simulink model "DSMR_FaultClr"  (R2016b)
settings: Solver=FixedStepDiscrete  StartTime=0.0  StopTime=10.0  FixedStep=0.01  RelTol=1e-3  EnableMultiTasking=on
undefined symbols (not defined in the file): bin2dec, DSMAUX_xClearTrg_C
libraries: simulink x156

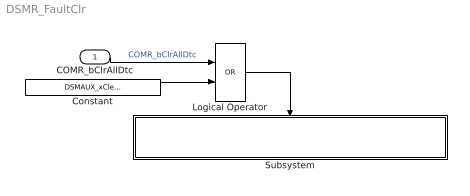
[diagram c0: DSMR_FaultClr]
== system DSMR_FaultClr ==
  COMR_bClrAllDtc : Inport
  Constant : Constant  Value=DSMAUX_xClearTrg_C
  Logical Operator : Logic  Operator=OR  AllPortsSameDT=off  OutDataTypeStr=boolean
  Subsystem : Subsystem
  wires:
  Constant/1 -> Logical Operator/2
  COMR_bClrAllDtc/1 -> Logical Operator/1  "COMR_bClrAllDtc"
  Logical Operator/1 -> Subsystem/Trigger

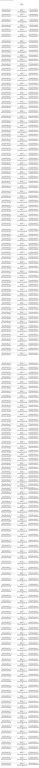
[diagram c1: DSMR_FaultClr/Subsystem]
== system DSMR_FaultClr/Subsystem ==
  Trigger : TriggerPort  VariantControl=Variant  PortDimensions=1
  Bitwise Operator{1..156} (156 alike) : simulink/Logic and Bit Operations/Bitwise Operator  logicop=AND  UseBitMask=on  BitMask=bin2dec('00000000')  BitMaskRealWorld=Stored Integer
  Data Store Read : DataStoreRead  DataStoreName=DFC_CurrRngErr
  Data Store Read1 : DataStoreRead  DataStoreName=DFC_BattVoltRngErr
  Data Store Read10 : DataStoreRead  DataStoreName=DFC_RcMsg2A3Mis
  Data Store Read100 : DataStoreRead  DataStoreName=DFC_CC2Chk
  Data Store Read101 : DataStoreRead  DataStoreName=DFC_APlusChk
  Data Store Read102 : DataStoreRead  DataStoreName=DFC_DChrgMsgTmt
  Data Store Read103 : DataStoreRead  DataStoreName=DFC_DChrgTNegElecMax
  Data Store Read104 : DataStoreRead  DataStoreName=DFC_DChrgTNegElecMin
  Data Store Read105 : DataStoreRead  DataStoreName=DFC_DChrgTNegElecSig
  Data Store Read106 : DataStoreRead  DataStoreName=DFC_DChrgTPosElecMax
  Data Store Read107 : DataStoreRead  DataStoreName=DFC_DChrgTPosElecMin
  Data Store Read108 : DataStoreRead  DataStoreName=DFC_DChrgTPosElecSig
  Data Store Read109 : DataStoreRead  DataStoreName=DFC_CcuSelfChkErr
  Data Store Read11 : DataStoreRead  DataStoreName=DFC_ChkSumMsg2A3Err
  Data Store Read110 : DataStoreRead  DataStoreName=DFC_ChrgOCMin
  Data Store Read111 : DataStoreRead  DataStoreName=DFC_ChrgOCMax
  Data Store Read112 : DataStoreRead  DataStoreName=DFC_DisChOCMax
  Data Store Read113 : DataStoreRead  DataStoreName=DFC_SocRngLoMax
  Data Store Read114 : DataStoreRead  DataStoreName=DFC_SocRngLoMin
  Data Store Read115 : DataStoreRead  DataStoreName=DFC_SocRngHiMax
  Data Store Read116 : DataStoreRead  DataStoreName=DFC_SocRngHiMin
  Data Store Read117 : DataStoreRead  DataStoreName=DFC_InClntOverTmp
  Data Store Read118 : DataStoreRead  DataStoreName=DFC_OutClntOverTmp
  Data Store Read119 : DataStoreRead  DataStoreName=DFC_ClntDsTElecMax
  Data Store Read12 : DataStoreRead  DataStoreName=DFC_RcMsg2A5Mis
  Data Store Read120 : DataStoreRead  DataStoreName=DFC_ClntDsTElecMin
  Data Store Read121 : DataStoreRead  DataStoreName=DFC_ClntDsTElecSig
  Data Store Read122 : DataStoreRead  DataStoreName=DFC_ClntUsTElecMax
  Data Store Read123 : DataStoreRead  DataStoreName=DFC_ClntUsTElecMin
  Data Store Read124 : DataStoreRead  DataStoreName=DFC_ClntUsTElecSig
  Data Store Read125 : DataStoreRead  DataStoreName=DFC_CoolPerfPlaus
  Data Store Read126 : DataStoreRead  DataStoreName=DFC_HtgPerfPlaus
  Data Store Read127 : DataStoreRead  DataStoreName=DFC_DChrgFobd
  Data Store Read128 : DataStoreRead  DataStoreName=DFC_DChrgHvOnFail
  Data Store Read129 : DataStoreRead  DataStoreName=DFC_AChgHVOnTmt
  Data Store Read13 : DataStoreRead  DataStoreName=DFC_RcMsg2A7Mis
  Data Store Read130 : DataStoreRead  DataStoreName=DFC_AChgHVOffTmt
  Data Store Read131 : DataStoreRead  DataStoreName=DFC_AChgS2ClsdTmt
  Data Store Read132 : DataStoreRead  DataStoreName=DFC_DChrgStakeErr
  Data Store Read133 : DataStoreRead  DataStoreName=DFC_DChrgStkVoltErr
  Data Store Read134 : DataStoreRead  DataStoreName=DFC_DChrgStkCurrErr
  Data Store Read135 : DataStoreRead  DataStoreName=DFC_AChgPileRdyTmt
  Data Store Read136 : DataStoreRead  DataStoreName=DFC_DChrgCHMTmt
  Data Store Read137 : DataStoreRead  DataStoreName=DFC_DChrgCRMTmt
  Data Store Read138 : DataStoreRead  DataStoreName=DFC_DChrgCMLTmt
  Data Store Read139 : DataStoreRead  DataStoreName=DFC_DChrgCROTmt
  Data Store Read14 : DataStoreRead  DataStoreName=DFC_MPosStuckMin
  Data Store Read140 : DataStoreRead  DataStoreName=DFC_DChrgCCSTmt
  Data Store Read141 : DataStoreRead  DataStoreName=DFC_DChrgCSTTmt
  Data Store Read142 : DataStoreRead  DataStoreName=DFC_DChrgCSDTmt
  Data Store Read143 : DataStoreRead  DataStoreName=DFC_DChrgParaChk
  Data Store Read144 : DataStoreRead  DataStoreName=DFC_DChrgCableChk
  Data Store Read145 : DataStoreRead  DataStoreName=DFC_DChrgSLACTOut
  Data Store Read146 : DataStoreRead  DataStoreName=DFC_DChrgCnntErr
  Data Store Read147 : DataStoreRead  DataStoreName=DFC_DChrgLckErr
  Data Store Read148 : DataStoreRead  DataStoreName=DFC_AChrgCnntErr
  Data Store Read149 : DataStoreRead  DataStoreName=DFC_AChgLckTmt
  Data Store Read15 : DataStoreRead  DataStoreName=DFC_MNegStuckMax
  Data Store Read150 : DataStoreRead  DataStoreName=DFC_AChgRdyPndiTmt
  Data Store Read151 : DataStoreRead  DataStoreName=DFC_AChgRdyTmt
  Data Store Read152 : DataStoreRead  DataStoreName=DFC_AChgingErr
  Data Store Read153 : DataStoreRead  DataStoreName=DFC_AChgUnlckTmt
  Data Store Read154 : DataStoreRead  DataStoreName=DFC_AChgFobd
  Data Store Read155 : DataStoreRead  DataStoreName=DFC_SocValJmp
  Data Store Read16 : DataStoreRead  DataStoreName=DFC_MNegStuckMin
  Data Store Read17 : DataStoreRead  DataStoreName=DFC_PrStuckMin
  Data Store Read18 : DataStoreRead  DataStoreName=DFC_CrashNpl
  Data Store Read19 : DataStoreRead  DataStoreName=DFC_FuseNpl
  Data Store Read2 : DataStoreRead  DataStoreName=DFC_BattHVMsgTmt
  Data Store Read20 : DataStoreRead  DataStoreName=DFC_Kl30cVoltLoErr
  Data Store Read21 : DataStoreRead  DataStoreName=DFC_PosStuckMax
  Data Store Read22 : DataStoreRead  DataStoreName=DFC_HvPwrUpFail
  Data Store Read23 : DataStoreRead  DataStoreName=DFC_DChrgPwrUpFail
  Data Store Read24 : DataStoreRead  DataStoreName=DFC_BattTAlrmMax
  Data Store Read25 : DataStoreRead  DataStoreName=DFC_BattTFaultMax
  Data Store Read26 : DataStoreRead  DataStoreName=DFC_DChrgPosStuckMax
  Data Store Read27 : DataStoreRead  DataStoreName=DFC_DChrgPosStuckMin
  Data Store Read28 : DataStoreRead  DataStoreName=DFC_DChrgNegStuckMax
  Data Store Read29 : DataStoreRead  DataStoreName=DFC_DChrgNegStuckMin
  Data Store Read3 : DataStoreRead  DataStoreName=DFC_BusHVMsgTmt
  Data Store Read30 : DataStoreRead  DataStoreName=DFC_BattTGradtMax
  Data Store Read31 : DataStoreRead  DataStoreName=DFC_CellVoltAlrmMax
  Data Store Read32 : DataStoreRead  DataStoreName=DFC_CellVoltFaultMax
  Data Store Read33 : DataStoreRead  DataStoreName=DFC_CellVoltFusfMax
  Data Store Read34 : DataStoreRead  DataStoreName=DFC_BattTAlrmMin
  Data Store Read35 : DataStoreRead  DataStoreName=DFC_BattTFaultMin
  Data Store Read36 : DataStoreRead  DataStoreName=DFC_BattTempVldMin
  Data Store Read37 : DataStoreRead  DataStoreName=DFC_BattTCnstMax
  Data Store Read38 : DataStoreRead  DataStoreName=DFC_CellVoltNpl
  Data Store Read39 : DataStoreRead  DataStoreName=DFC_Msg2E6Tmt
  Data Store Read4 : DataStoreRead  DataStoreName=DFC_638LinCommErr
  Data Store Read40 : DataStoreRead  DataStoreName=DFC_RcMsg2E0Mis
  Data Store Read41 : DataStoreRead  DataStoreName=DFC_ChkSumMsg2E0Err
  Data Store Read42 : DataStoreRead  DataStoreName=DFC_CellVoltAlrmMin
  Data Store Read43 : DataStoreRead  DataStoreName=DFC_CellVoltFusfMin
  Data Store Read44 : DataStoreRead  DataStoreName=DFC_CellVoltFaultMin
  Data Store Read45 : DataStoreRead  DataStoreName=DFC_CellVoltVldMin
  Data Store Read46 : DataStoreRead  DataStoreName=DFC_ChrgOCNpl
  Data Store Read47 : DataStoreRead  DataStoreName=DFC_DisChOCNpl
  Data Store Read48 : DataStoreRead  DataStoreName=DFC_BattVoltHiMax
  Data Store Read49 : DataStoreRead  DataStoreName=DFC_BattVoltLoMin
  Data Store Read5 : DataStoreRead  DataStoreName=DFC_CellTempTmt
  Data Store Read50 : DataStoreRead  DataStoreName=DFC_RcMsg2E1Mis
  Data Store Read51 : DataStoreRead  DataStoreName=DFC_ChkSumMsg2E1Err
  Data Store Read52 : DataStoreRead  DataStoreName=DFC_DcCanBusOff
  Data Store Read53 : DataStoreRead  DataStoreName=DFC_DChrgTCnntMax
  Data Store Read54 : DataStoreRead  DataStoreName=DFC_CurrChrgPlaus
  Data Store Read55 : DataStoreRead  DataStoreName=DFC_BattUNpl
  Data Store Read56 : DataStoreRead  DataStoreName=DFC_BattVoltVld
  Data Store Read57 : DataStoreRead  DataStoreName=DFC_PackUNpl
  Data Store Read58 : DataStoreRead  DataStoreName=DFC_ThmRnwy
  Data Store Read59 : DataStoreRead  DataStoreName=DFC_AChrgPortOvrTemp
  Data Store Read6 : DataStoreRead  DataStoreName=DFC_CellVoltTmt
  Data Store Read60 : DataStoreRead  DataStoreName=DFC_CurrOffsPlaus
  Data Store Read61 : DataStoreRead  DataStoreName=DFC_CurrStukPlaus
  Data Store Read62 : DataStoreRead  DataStoreName=DFC_EepReadErr
  Data Store Read63 : DataStoreRead  DataStoreName=DFC_BalStuckMax
  Data Store Read64 : DataStoreRead  DataStoreName=DFC_DChrgVoltVld
  Data Store Read65 : DataStoreRead  DataStoreName=DFC_BoardTempTmt
  Data Store Read66 : DataStoreRead  DataStoreName=DFC_PackVoltVld
  Data Store Read67 : DataStoreRead  DataStoreName=DFC_BalStuckMin
  Data Store Read68 : DataStoreRead  DataStoreName=DFC_CSCPwrSpyHiErr
  Data Store Read69 : DataStoreRead  DataStoreName=DFC_DChrgUNpl
  Data Store Read7 : DataStoreRead  DataStoreName=DFC_InCanBusOff
  Data Store Read70 : DataStoreRead  DataStoreName=DFC_HvilMax
  Data Store Read71 : DataStoreRead  DataStoreName=DFC_HvilMin
  Data Store Read72 : DataStoreRead  DataStoreName=DFC_HvilSig
  Data Store Read73 : DataStoreRead  DataStoreName=DFC_ChkSumMsg050Err
  Data Store Read74 : DataStoreRead  DataStoreName=DFC_RcMsg050Mis
  Data Store Read75 : DataStoreRead  DataStoreName=DFC_CrashHwNpl
  Data Store Read76 : DataStoreRead  DataStoreName=DFC_IsoChkLv1
  Data Store Read77 : DataStoreRead  DataStoreName=DFC_IsoChkLv2
  Data Store Read78 : DataStoreRead  DataStoreName=DFC_DisChOCMin
  Data Store Read79 : DataStoreRead  DataStoreName=DFC_InsResValdFault
  Data Store Read8 : DataStoreRead  DataStoreName=DFC_VeCanBusOff
  Data Store Read80 : DataStoreRead  DataStoreName=DFC_Kl30OutRngErr
  Data Store Read81 : DataStoreRead  DataStoreName=DFC_Kl30VoltLoErr
  Data Store Read82 : DataStoreRead  DataStoreName=DFC_Kl30VoltHiErr
  Data Store Read83 : DataStoreRead  DataStoreName=DFC_CSCPwrSpyLoErr
  Data Store Read84 : DataStoreRead  DataStoreName=DFC_CmcBordOTMax
  Data Store Read85 : DataStoreRead  DataStoreName=DFC_BattTWarnMax
  Data Store Read86 : DataStoreRead  DataStoreName=DFC_BattTWarnMin
  Data Store Read87 : DataStoreRead  DataStoreName=DFC_BattTempVldMax
  Data Store Read88 : DataStoreRead  DataStoreName=DFC_BattTHopMax
  Data Store Read89 : DataStoreRead  DataStoreName=DFC_CellVoltRngHiErr
  Data Store Read9 : DataStoreRead  DataStoreName=DFC_Msg2A3Tmt
  Data Store Read90 : DataStoreRead  DataStoreName=DFC_CellVoltRngLoErr
  Data Store Read91 : DataStoreRead  DataStoreName=DFC_CellVoltWarnMax
  Data Store Read92 : DataStoreRead  DataStoreName=DFC_CellVoltWarnMin
  Data Store Read93 : DataStoreRead  DataStoreName=DFC_CellVoltVldMax
  Data Store Read94 : DataStoreRead  DataStoreName=DFC_AChrgCurrMish
  Data Store Read95 : DataStoreRead  DataStoreName=DFC_DChrgCurrMish
  Data Store Read96 : DataStoreRead  DataStoreName=DFC_DChrgLowTempCurrMish
  Data Store Read97 : DataStoreRead  DataStoreName=DFC_AChrgVoltMish
  Data Store Read98 : DataStoreRead  DataStoreName=DFC_DChrgVoltMish
  Data Store Read99 : DataStoreRead  DataStoreName=DFC_DChrgBattTMin
  Data Store Write : DataStoreWrite  DataStoreName=DFC_CurrRngErr
  Data Store Write1 : DataStoreWrite  DataStoreName=DFC_BattVoltRngErr
  Data Store Write10 : DataStoreWrite  DataStoreName=DFC_RcMsg2A3Mis
  Data Store Write100 : DataStoreWrite  DataStoreName=DFC_CC2Chk
  Data Store Write101 : DataStoreWrite  DataStoreName=DFC_APlusChk
  Data Store Write102 : DataStoreWrite  DataStoreName=DFC_DChrgMsgTmt
  Data Store Write103 : DataStoreWrite  DataStoreName=DFC_DChrgTNegElecMax
  Data Store Write104 : DataStoreWrite  DataStoreName=DFC_DChrgTNegElecMin
  Data Store Write105 : DataStoreWrite  DataStoreName=DFC_DChrgTNegElecSig
  Data Store Write106 : DataStoreWrite  DataStoreName=DFC_DChrgTPosElecMax
  Data Store Write107 : DataStoreWrite  DataStoreName=DFC_DChrgTPosElecMin
  Data Store Write108 : DataStoreWrite  DataStoreName=DFC_DChrgTPosElecSig
  Data Store Write109 : DataStoreWrite  DataStoreName=DFC_CcuSelfChkErr
  Data Store Write11 : DataStoreWrite  DataStoreName=DFC_ChkSumMsg2A3Err
  Data Store Write110 : DataStoreWrite  DataStoreName=DFC_ChrgOCMin
  Data Store Write111 : DataStoreWrite  DataStoreName=DFC_ChrgOCMax
  Data Store Write112 : DataStoreWrite  DataStoreName=DFC_DisChOCMax
  Data Store Write113 : DataStoreWrite  DataStoreName=DFC_SocRngLoMax
  Data Store Write114 : DataStoreWrite  DataStoreName=DFC_SocRngLoMin
  Data Store Write115 : DataStoreWrite  DataStoreName=DFC_SocRngHiMax
  Data Store Write116 : DataStoreWrite  DataStoreName=DFC_SocRngHiMin
  Data Store Write117 : DataStoreWrite  DataStoreName=DFC_InClntOverTmp
  Data Store Write118 : DataStoreWrite  DataStoreName=DFC_OutClntOverTmp
  Data Store Write119 : DataStoreWrite  DataStoreName=DFC_ClntDsTElecMax
  Data Store Write12 : DataStoreWrite  DataStoreName=DFC_RcMsg2A5Mis
  Data Store Write120 : DataStoreWrite  DataStoreName=DFC_ClntDsTElecMin
  Data Store Write121 : DataStoreWrite  DataStoreName=DFC_ClntDsTElecSig
  Data Store Write122 : DataStoreWrite  DataStoreName=DFC_ClntUsTElecMax
  Data Store Write123 : DataStoreWrite  DataStoreName=DFC_ClntUsTElecMin
  Data Store Write124 : DataStoreWrite  DataStoreName=DFC_ClntUsTElecSig
  Data Store Write125 : DataStoreWrite  DataStoreName=DFC_CoolPerfPlaus
  Data Store Write126 : DataStoreWrite  DataStoreName=DFC_HtgPerfPlaus
  Data Store Write127 : DataStoreWrite  DataStoreName=DFC_DChrgFobd
  Data Store Write128 : DataStoreWrite  DataStoreName=DFC_DChrgHvOnFail
  Data Store Write129 : DataStoreWrite  DataStoreName=DFC_AChgHVOnTmt
  Data Store Write13 : DataStoreWrite  DataStoreName=DFC_RcMsg2A7Mis
  Data Store Write130 : DataStoreWrite  DataStoreName=DFC_AChgHVOffTmt
  Data Store Write131 : DataStoreWrite  DataStoreName=DFC_AChgS2ClsdTmt
  Data Store Write132 : DataStoreWrite  DataStoreName=DFC_DChrgStakeErr
  Data Store Write133 : DataStoreWrite  DataStoreName=DFC_DChrgStkVoltErr
  Data Store Write134 : DataStoreWrite  DataStoreName=DFC_DChrgStkCurrErr
  Data Store Write135 : DataStoreWrite  DataStoreName=DFC_AChgPileRdyTmt
  Data Store Write136 : DataStoreWrite  DataStoreName=DFC_DChrgCHMTmt
  Data Store Write137 : DataStoreWrite  DataStoreName=DFC_DChrgCRMTmt
  Data Store Write138 : DataStoreWrite  DataStoreName=DFC_DChrgCMLTmt
  Data Store Write139 : DataStoreWrite  DataStoreName=DFC_DChrgCROTmt
  Data Store Write14 : DataStoreWrite  DataStoreName=DFC_MPosStuckMin
  Data Store Write140 : DataStoreWrite  DataStoreName=DFC_DChrgCCSTmt
  Data Store Write141 : DataStoreWrite  DataStoreName=DFC_DChrgCSTTmt
  Data Store Write142 : DataStoreWrite  DataStoreName=DFC_DChrgCSDTmt
  Data Store Write143 : DataStoreWrite  DataStoreName=DFC_DChrgParaChk
  Data Store Write144 : DataStoreWrite  DataStoreName=DFC_DChrgCableChk
  Data Store Write145 : DataStoreWrite  DataStoreName=DFC_DChrgSLACTOut
  Data Store Write146 : DataStoreWrite  DataStoreName=DFC_DChrgCnntErr
  Data Store Write147 : DataStoreWrite  DataStoreName=DFC_DChrgLckErr
  Data Store Write148 : DataStoreWrite  DataStoreName=DFC_AChrgCnntErr
  Data Store Write149 : DataStoreWrite  DataStoreName=DFC_AChgLckTmt
  Data Store Write15 : DataStoreWrite  DataStoreName=DFC_MNegStuckMax
  Data Store Write150 : DataStoreWrite  DataStoreName=DFC_AChgRdyPndiTmt
  Data Store Write151 : DataStoreWrite  DataStoreName=DFC_AChgRdyTmt
  Data Store Write152 : DataStoreWrite  DataStoreName=DFC_AChgingErr
  Data Store Write153 : DataStoreWrite  DataStoreName=DFC_AChgUnlckTmt
  Data Store Write154 : DataStoreWrite  DataStoreName=DFC_AChgFobd
  Data Store Write155 : DataStoreWrite  DataStoreName=DFC_SocValJmp
  Data Store Write16 : DataStoreWrite  DataStoreName=DFC_MNegStuckMin
  Data Store Write17 : DataStoreWrite  DataStoreName=DFC_PrStuckMin
  Data Store Write18 : DataStoreWrite  DataStoreName=DFC_CrashNpl
  Data Store Write19 : DataStoreWrite  DataStoreName=DFC_FuseNpl
  Data Store Write2 : DataStoreWrite  DataStoreName=DFC_BattHVMsgTmt
  Data Store Write20 : DataStoreWrite  DataStoreName=DFC_Kl30cVoltLoErr
  Data Store Write21 : DataStoreWrite  DataStoreName=DFC_PosStuckMax
  Data Store Write22 : DataStoreWrite  DataStoreName=DFC_HvPwrUpFail
  Data Store Write23 : DataStoreWrite  DataStoreName=DFC_DChrgPwrUpFail
  Data Store Write24 : DataStoreWrite  DataStoreName=DFC_BattTAlrmMax
  Data Store Write25 : DataStoreWrite  DataStoreName=DFC_BattTFaultMax
  Data Store Write26 : DataStoreWrite  DataStoreName=DFC_DChrgPosStuckMax
  Data Store Write27 : DataStoreWrite  DataStoreName=DFC_DChrgPosStuckMin
  Data Store Write28 : DataStoreWrite  DataStoreName=DFC_DChrgNegStuckMax
  Data Store Write29 : DataStoreWrite  DataStoreName=DFC_DChrgNegStuckMin
  Data Store Write3 : DataStoreWrite  DataStoreName=DFC_BusHVMsgTmt
  Data Store Write30 : DataStoreWrite  DataStoreName=DFC_BattTGradtMax
  Data Store Write31 : DataStoreWrite  DataStoreName=DFC_CellVoltAlrmMax
  Data Store Write32 : DataStoreWrite  DataStoreName=DFC_CellVoltFaultMax
  Data Store Write33 : DataStoreWrite  DataStoreName=DFC_CellVoltFusfMax
  Data Store Write34 : DataStoreWrite  DataStoreName=DFC_BattTAlrmMin
  Data Store Write35 : DataStoreWrite  DataStoreName=DFC_BattTFaultMin
  Data Store Write36 : DataStoreWrite  DataStoreName=DFC_BattTempVldMin
  Data Store Write37 : DataStoreWrite  DataStoreName=DFC_BattTCnstMax
  Data Store Write38 : DataStoreWrite  DataStoreName=DFC_CellVoltNpl
  Data Store Write39 : DataStoreWrite  DataStoreName=DFC_Msg2E6Tmt
  Data Store Write4 : DataStoreWrite  DataStoreName=DFC_638LinCommErr
  Data Store Write40 : DataStoreWrite  DataStoreName=DFC_RcMsg2E0Mis
  Data Store Write41 : DataStoreWrite  DataStoreName=DFC_ChkSumMsg2E0Err
  Data Store Write42 : DataStoreWrite  DataStoreName=DFC_CellVoltAlrmMin
  Data Store Write43 : DataStoreWrite  DataStoreName=DFC_CellVoltFusfMin
  Data Store Write44 : DataStoreWrite  DataStoreName=DFC_CellVoltFaultMin
  Data Store Write45 : DataStoreWrite  DataStoreName=DFC_CellVoltVldMin
  Data Store Write46 : DataStoreWrite  DataStoreName=DFC_ChrgOCNpl
  Data Store Write47 : DataStoreWrite  DataStoreName=DFC_DisChOCNpl
  Data Store Write48 : DataStoreWrite  DataStoreName=DFC_BattVoltHiMax
  Data Store Write49 : DataStoreWrite  DataStoreName=DFC_BattVoltLoMin
  Data Store Write5 : DataStoreWrite  DataStoreName=DFC_CellTempTmt
  Data Store Write50 : DataStoreWrite  DataStoreName=DFC_RcMsg2E1Mis
  Data Store Write51 : DataStoreWrite  DataStoreName=DFC_ChkSumMsg2E1Err
  Data Store Write52 : DataStoreWrite  DataStoreName=DFC_DcCanBusOff
  Data Store Write53 : DataStoreWrite  DataStoreName=DFC_DChrgTCnntMax
  Data Store Write54 : DataStoreWrite  DataStoreName=DFC_CurrChrgPlaus
  Data Store Write55 : DataStoreWrite  DataStoreName=DFC_BattUNpl
  Data Store Write56 : DataStoreWrite  DataStoreName=DFC_BattVoltVld
  Data Store Write57 : DataStoreWrite  DataStoreName=DFC_PackUNpl
  Data Store Write58 : DataStoreWrite  DataStoreName=DFC_ThmRnwy
  Data Store Write59 : DataStoreWrite  DataStoreName=DFC_AChrgPortOvrTemp
  Data Store Write6 : DataStoreWrite  DataStoreName=DFC_CellVoltTmt
  Data Store Write60 : DataStoreWrite  DataStoreName=DFC_CurrOffsPlaus
  Data Store Write61 : DataStoreWrite  DataStoreName=DFC_CurrStukPlaus
  Data Store Write62 : DataStoreWrite  DataStoreName=DFC_EepReadErr
  Data Store Write63 : DataStoreWrite  DataStoreName=DFC_BalStuckMax
  Data Store Write64 : DataStoreWrite  DataStoreName=DFC_DChrgVoltVld
  Data Store Write65 : DataStoreWrite  DataStoreName=DFC_BoardTempTmt
  Data Store Write66 : DataStoreWrite  DataStoreName=DFC_PackVoltVld
  Data Store Write67 : DataStoreWrite  DataStoreName=DFC_BalStuckMin
  Data Store Write68 : DataStoreWrite  DataStoreName=DFC_CSCPwrSpyHiErr
  Data Store Write69 : DataStoreWrite  DataStoreName=DFC_DChrgUNpl
  Data Store Write7 : DataStoreWrite  DataStoreName=DFC_InCanBusOff
  Data Store Write70 : DataStoreWrite  DataStoreName=DFC_HvilMax
  Data Store Write71 : DataStoreWrite  DataStoreName=DFC_HvilMin
  Data Store Write72 : DataStoreWrite  DataStoreName=DFC_HvilSig
  Data Store Write73 : DataStoreWrite  DataStoreName=DFC_ChkSumMsg050Err
  Data Store Write74 : DataStoreWrite  DataStoreName=DFC_RcMsg050Mis
  Data Store Write75 : DataStoreWrite  DataStoreName=DFC_CrashHwNpl
  Data Store Write76 : DataStoreWrite  DataStoreName=DFC_IsoChkLv1
  Data Store Write77 : DataStoreWrite  DataStoreName=DFC_IsoChkLv2
  Data Store Write78 : DataStoreWrite  DataStoreName=DFC_DisChOCMin
  Data Store Write79 : DataStoreWrite  DataStoreName=DFC_InsResValdFault
  Data Store Write8 : DataStoreWrite  DataStoreName=DFC_VeCanBusOff
  Data Store Write80 : DataStoreWrite  DataStoreName=DFC_Kl30OutRngErr
  Data Store Write81 : DataStoreWrite  DataStoreName=DFC_Kl30VoltLoErr
  Data Store Write82 : DataStoreWrite  DataStoreName=DFC_Kl30VoltHiErr
  Data Store Write83 : DataStoreWrite  DataStoreName=DFC_CSCPwrSpyLoErr
  Data Store Write84 : DataStoreWrite  DataStoreName=DFC_CmcBordOTMax
  Data Store Write85 : DataStoreWrite  DataStoreName=DFC_BattTWarnMax
  Data Store Write86 : DataStoreWrite  DataStoreName=DFC_BattTWarnMin
  Data Store Write87 : DataStoreWrite  DataStoreName=DFC_BattTempVldMax
  Data Store Write88 : DataStoreWrite  DataStoreName=DFC_BattTHopMax
  Data Store Write89 : DataStoreWrite  DataStoreName=DFC_CellVoltRngHiErr
  Data Store Write9 : DataStoreWrite  DataStoreName=DFC_Msg2A3Tmt
  Data Store Write90 : DataStoreWrite  DataStoreName=DFC_CellVoltRngLoErr
  Data Store Write91 : DataStoreWrite  DataStoreName=DFC_CellVoltWarnMax
  Data Store Write92 : DataStoreWrite  DataStoreName=DFC_CellVoltWarnMin
  Data Store Write93 : DataStoreWrite  DataStoreName=DFC_CellVoltVldMax
  Data Store Write94 : DataStoreWrite  DataStoreName=DFC_AChrgCurrMish
  Data Store Write95 : DataStoreWrite  DataStoreName=DFC_DChrgCurrMish
  Data Store Write96 : DataStoreWrite  DataStoreName=DFC_DChrgLowTempCurrMish
  Data Store Write97 : DataStoreWrite  DataStoreName=DFC_AChrgVoltMish
  Data Store Write98 : DataStoreWrite  DataStoreName=DFC_DChrgVoltMish
  Data Store Write99 : DataStoreWrite  DataStoreName=DFC_DChrgBattTMin
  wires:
  Data Store Read1/1 -> Bitwise Operator2/1
  Bitwise Operator2/1 -> Data Store Write1/1
  Data Store Read2/1 -> Bitwise Operator3/1
  Bitwise Operator3/1 -> Data Store Write2/1
  Data Store Read3/1 -> Bitwise Operator4/1
  Bitwise Operator4/1 -> Data Store Write3/1
  Data Store Read4/1 -> Bitwise Operator5/1
  Bitwise Operator5/1 -> Data Store Write4/1
  Data Store Read5/1 -> Bitwise Operator6/1
  Bitwise Operator6/1 -> Data Store Write5/1
  Data Store Read6/1 -> Bitwise Operator7/1
  Bitwise Operator7/1 -> Data Store Write6/1
  Data Store Read7/1 -> Bitwise Operator8/1
  Bitwise Operator8/1 -> Data Store Write7/1
  Data Store Read8/1 -> Bitwise Operator9/1
  Bitwise Operator9/1 -> Data Store Write8/1
  Data Store Read9/1 -> Bitwise Operator10/1
  Bitwise Operator10/1 -> Data Store Write9/1
  Data Store Read10/1 -> Bitwise Operator11/1
  Bitwise Operator11/1 -> Data Store Write10/1
  Data Store Read11/1 -> Bitwise Operator12/1
  Bitwise Operator12/1 -> Data Store Write11/1
  Data Store Read12/1 -> Bitwise Operator13/1
  Bitwise Operator13/1 -> Data Store Write12/1
  Data Store Read13/1 -> Bitwise Operator14/1
  Bitwise Operator14/1 -> Data Store Write13/1
  Data Store Read18/1 -> Bitwise Operator15/1
  Bitwise Operator15/1 -> Data Store Write18/1
  Data Store Read19/1 -> Bitwise Operator16/1
  Bitwise Operator16/1 -> Data Store Write19/1
  Data Store Read20/1 -> Bitwise Operator17/1
  Bitwise Operator17/1 -> Data Store Write20/1
  Data Store Read21/1 -> Bitwise Operator18/1
  Bitwise Operator18/1 -> Data Store Write21/1
  Data Store Read14/1 -> Bitwise Operator19/1
  Bitwise Operator19/1 -> Data Store Write14/1
  Data Store Read15/1 -> Bitwise Operator20/1
  Bitwise Operator20/1 -> Data Store Write15/1
  Data Store Read16/1 -> Bitwise Operator21/1
  Bitwise Operator21/1 -> Data Store Write16/1
  Data Store Read17/1 -> Bitwise Operator22/1
  Bitwise Operator22/1 -> Data Store Write17/1
  Data Store Read26/1 -> Bitwise Operator23/1
  Bitwise Operator23/1 -> Data Store Write26/1
  Data Store Read27/1 -> Bitwise Operator24/1
  Bitwise Operator24/1 -> Data Store Write27/1
  Data Store Read28/1 -> Bitwise Operator25/1
  Bitwise Operator25/1 -> Data Store Write28/1
  Data Store Read29/1 -> Bitwise Operator26/1
  Bitwise Operator26/1 -> Data Store Write29/1
  Data Store Read22/1 -> Bitwise Operator27/1
  Bitwise Operator27/1 -> Data Store Write22/1
  Data Store Read23/1 -> Bitwise Operator28/1
  Bitwise Operator28/1 -> Data Store Write23/1
  Data Store Read24/1 -> Bitwise Operator29/1
  Bitwise Operator29/1 -> Data Store Write24/1
  Data Store Read25/1 -> Bitwise Operator30/1
  Bitwise Operator30/1 -> Data Store Write25/1
  Data Store Read34/1 -> Bitwise Operator31/1
  Bitwise Operator31/1 -> Data Store Write34/1
  Data Store Read35/1 -> Bitwise Operator32/1
  Bitwise Operator32/1 -> Data Store Write35/1
  Data Store Read36/1 -> Bitwise Operator33/1
  Bitwise Operator33/1 -> Data Store Write36/1
  Data Store Read37/1 -> Bitwise Operator34/1
  Bitwise Operator34/1 -> Data Store Write37/1
  Data Store Read30/1 -> Bitwise Operator35/1
  Bitwise Operator35/1 -> Data Store Write30/1
  Data Store Read31/1 -> Bitwise Operator36/1
  Bitwise Operator36/1 -> Data Store Write31/1
  Data Store Read32/1 -> Bitwise Operator37/1
  Bitwise Operator37/1 -> Data Store Write32/1
  Data Store Read33/1 -> Bitwise Operator38/1
  Bitwise Operator38/1 -> Data Store Write33/1
  Data Store Read42/1 -> Bitwise Operator39/1
  Bitwise Operator39/1 -> Data Store Write42/1
  Data Store Read43/1 -> Bitwise Operator40/1
  Bitwise Operator40/1 -> Data Store Write43/1
  Data Store Read44/1 -> Bitwise Operator41/1
  Bitwise Operator41/1 -> Data Store Write44/1
  Data Store Read45/1 -> Bitwise Operator42/1
  Bitwise Operator42/1 -> Data Store Write45/1
  Data Store Read38/1 -> Bitwise Operator43/1
  Bitwise Operator43/1 -> Data Store Write38/1
  Data Store Read39/1 -> Bitwise Operator44/1
  Bitwise Operator44/1 -> Data Store Write39/1
  Data Store Read40/1 -> Bitwise Operator45/1
  Bitwise Operator45/1 -> Data Store Write40/1
  Data Store Read41/1 -> Bitwise Operator46/1
  Bitwise Operator46/1 -> Data Store Write41/1
  Data Store Read50/1 -> Bitwise Operator47/1
  Bitwise Operator47/1 -> Data Store Write50/1
  Data Store Read51/1 -> Bitwise Operator48/1
  Bitwise Operator48/1 -> Data Store Write51/1
  Data Store Read52/1 -> Bitwise Operator49/1
  Bitwise Operator49/1 -> Data Store Write52/1
  Data Store Read53/1 -> Bitwise Operator50/1
  Bitwise Operator50/1 -> Data Store Write53/1
  Data Store Read46/1 -> Bitwise Operator51/1
  Bitwise Operator51/1 -> Data Store Write46/1
  Data Store Read47/1 -> Bitwise Operator52/1
  Bitwise Operator52/1 -> Data Store Write47/1
  Data Store Read48/1 -> Bitwise Operator53/1
  Bitwise Operator53/1 -> Data Store Write48/1
  Data Store Read49/1 -> Bitwise Operator54/1
  Bitwise Operator54/1 -> Data Store Write49/1
  Data Store Read58/1 -> Bitwise Operator55/1
  Bitwise Operator55/1 -> Data Store Write58/1
  Data Store Read59/1 -> Bitwise Operator56/1
  Bitwise Operator56/1 -> Data Store Write59/1
  Data Store Read60/1 -> Bitwise Operator57/1
  Bitwise Operator57/1 -> Data Store Write60/1
  Data Store Read61/1 -> Bitwise Operator58/1
  Bitwise Operator58/1 -> Data Store Write61/1
  Data Store Read54/1 -> Bitwise Operator59/1
  Bitwise Operator59/1 -> Data Store Write54/1
  Data Store Read55/1 -> Bitwise Operator60/1
  Bitwise Operator60/1 -> Data Store Write55/1
  Data Store Read56/1 -> Bitwise Operator61/1
  Bitwise Operator61/1 -> Data Store Write56/1
  Data Store Read57/1 -> Bitwise Operator62/1
  Bitwise Operator62/1 -> Data Store Write57/1
  Data Store Read66/1 -> Bitwise Operator63/1
  Bitwise Operator63/1 -> Data Store Write66/1
  Data Store Read69/1 -> Bitwise Operator64/1
  Bitwise Operator64/1 -> Data Store Write69/1
  Data Store Read64/1 -> Bitwise Operator65/1
  Bitwise Operator65/1 -> Data Store Write64/1
  Data Store Read65/1 -> Bitwise Operator66/1
  Bitwise Operator66/1 -> Data Store Write65/1
  Data Store Read70/1 -> Bitwise Operator67/1
  Bitwise Operator67/1 -> Data Store Write70/1
  Data Store Read71/1 -> Bitwise Operator68/1
  Bitwise Operator68/1 -> Data Store Write71/1
  Data Store Read72/1 -> Bitwise Operator69/1
  Bitwise Operator69/1 -> Data Store Write72/1
  Data Store Read73/1 -> Bitwise Operator70/1
  Bitwise Operator70/1 -> Data Store Write73/1
  Data Store Read74/1 -> Bitwise Operator71/1
  Bitwise Operator71/1 -> Data Store Write74/1
  Data Store Read75/1 -> Bitwise Operator72/1
  Bitwise Operator72/1 -> Data Store Write75/1
  Data Store Read76/1 -> Bitwise Operator73/1
  Bitwise Operator73/1 -> Data Store Write76/1
  Data Store Read77/1 -> Bitwise Operator74/1
  Bitwise Operator74/1 -> Data Store Write77/1
  Data Store Read79/1 -> Bitwise Operator76/1
  Bitwise Operator76/1 -> Data Store Write79/1
  Data Store Read80/1 -> Bitwise Operator77/1
  Bitwise Operator77/1 -> Data Store Write80/1
  Data Store Read81/1 -> Bitwise Operator78/1
  Bitwise Operator78/1 -> Data Store Write81/1
  Data Store Read82/1 -> Bitwise Operator79/1
  Bitwise Operator79/1 -> Data Store Write82/1
  Data Store Read/1 -> Bitwise Operator1/1
  Bitwise Operator1/1 -> Data Store Write/1
  Data Store Read62/1 -> Bitwise Operator80/1
  Bitwise Operator80/1 -> Data Store Write62/1
  Data Store Read63/1 -> Bitwise Operator81/1
  Bitwise Operator81/1 -> Data Store Write63/1
  Data Store Read67/1 -> Bitwise Operator82/1
  Bitwise Operator82/1 -> Data Store Write67/1
  Data Store Read68/1 -> Bitwise Operator83/1
  Bitwise Operator83/1 -> Data Store Write68/1
  Data Store Read83/1 -> Bitwise Operator84/1
  Bitwise Operator84/1 -> Data Store Write83/1
  Data Store Read84/1 -> Bitwise Operator87/1
  Bitwise Operator87/1 -> Data Store Write84/1
  Data Store Read85/1 -> Bitwise Operator85/1
  Bitwise Operator85/1 -> Data Store Write85/1
  Data Store Read86/1 -> Bitwise Operator86/1
  Bitwise Operator86/1 -> Data Store Write86/1
  Data Store Read87/1 -> Bitwise Operator88/1
  Bitwise Operator88/1 -> Data Store Write87/1
  Data Store Read88/1 -> Bitwise Operator89/1
  Bitwise Operator89/1 -> Data Store Write88/1
  Data Store Read89/1 -> Bitwise Operator90/1
  Bitwise Operator90/1 -> Data Store Write89/1
  Data Store Read90/1 -> Bitwise Operator91/1
  Bitwise Operator91/1 -> Data Store Write90/1
  Data Store Read91/1 -> Bitwise Operator92/1
  Bitwise Operator92/1 -> Data Store Write91/1
  Data Store Read92/1 -> Bitwise Operator93/1
  Bitwise Operator93/1 -> Data Store Write92/1
  Data Store Read93/1 -> Bitwise Operator94/1
  Bitwise Operator94/1 -> Data Store Write93/1
  Data Store Read94/1 -> Bitwise Operator95/1
  Bitwise Operator95/1 -> Data Store Write94/1
  Data Store Read95/1 -> Bitwise Operator96/1
  Bitwise Operator96/1 -> Data Store Write95/1
  Data Store Read96/1 -> Bitwise Operator97/1
  Bitwise Operator97/1 -> Data Store Write96/1
  Data Store Read97/1 -> Bitwise Operator98/1
  Bitwise Operator98/1 -> Data Store Write97/1
  Data Store Read98/1 -> Bitwise Operator99/1
  Bitwise Operator99/1 -> Data Store Write98/1
  Data Store Read99/1 -> Bitwise Operator100/1
  Bitwise Operator100/1 -> Data Store Write99/1
  Data Store Read100/1 -> Bitwise Operator101/1
  Bitwise Operator101/1 -> Data Store Write100/1
  Data Store Read101/1 -> Bitwise Operator102/1
  Bitwise Operator102/1 -> Data Store Write101/1
  Data Store Read102/1 -> Bitwise Operator103/1
  Bitwise Operator103/1 -> Data Store Write102/1
  Data Store Read103/1 -> Bitwise Operator104/1
  Bitwise Operator104/1 -> Data Store Write103/1
  Data Store Read104/1 -> Bitwise Operator105/1
  Bitwise Operator105/1 -> Data Store Write104/1
  Data Store Read105/1 -> Bitwise Operator106/1
  Bitwise Operator106/1 -> Data Store Write105/1
  Data Store Read106/1 -> Bitwise Operator107/1
  Bitwise Operator107/1 -> Data Store Write106/1
  Data Store Read107/1 -> Bitwise Operator108/1
  Bitwise Operator108/1 -> Data Store Write107/1
  Data Store Read108/1 -> Bitwise Operator109/1
  Bitwise Operator109/1 -> Data Store Write108/1
  Data Store Read109/1 -> Bitwise Operator110/1
  Bitwise Operator110/1 -> Data Store Write109/1
  Data Store Read110/1 -> Bitwise Operator111/1
  Bitwise Operator111/1 -> Data Store Write110/1
  Data Store Read111/1 -> Bitwise Operator112/1
  Bitwise Operator112/1 -> Data Store Write111/1
  Data Store Read78/1 -> Bitwise Operator75/1
  Bitwise Operator75/1 -> Data Store Write78/1
  Data Store Read112/1 -> Bitwise Operator113/1
  Bitwise Operator113/1 -> Data Store Write112/1
  Data Store Read113/1 -> Bitwise Operator114/1
  Bitwise Operator114/1 -> Data Store Write113/1
  Data Store Read114/1 -> Bitwise Operator115/1
  Bitwise Operator115/1 -> Data Store Write114/1
  Data Store Read115/1 -> Bitwise Operator116/1
  Bitwise Operator116/1 -> Data Store Write115/1
  Data Store Read116/1 -> Bitwise Operator117/1
  Bitwise Operator117/1 -> Data Store Write116/1
  Data Store Read117/1 -> Bitwise Operator118/1
  Bitwise Operator118/1 -> Data Store Write117/1
  Data Store Read118/1 -> Bitwise Operator119/1
  Bitwise Operator119/1 -> Data Store Write118/1
  Data Store Read119/1 -> Bitwise Operator120/1
  Bitwise Operator120/1 -> Data Store Write119/1
  Data Store Read120/1 -> Bitwise Operator121/1
  Bitwise Operator121/1 -> Data Store Write120/1
  Data Store Read121/1 -> Bitwise Operator122/1
  Bitwise Operator122/1 -> Data Store Write121/1
  Data Store Read122/1 -> Bitwise Operator123/1
  Bitwise Operator123/1 -> Data Store Write122/1
  Data Store Read123/1 -> Bitwise Operator124/1
  Bitwise Operator124/1 -> Data Store Write123/1
  Data Store Read124/1 -> Bitwise Operator125/1
  Bitwise Operator125/1 -> Data Store Write124/1
  Data Store Read125/1 -> Bitwise Operator126/1
  Bitwise Operator126/1 -> Data Store Write125/1
  Data Store Read126/1 -> Bitwise Operator127/1
  Bitwise Operator127/1 -> Data Store Write126/1
  Data Store Read127/1 -> Bitwise Operator128/1
  Bitwise Operator128/1 -> Data Store Write127/1
  Data Store Read128/1 -> Bitwise Operator129/1
  Bitwise Operator129/1 -> Data Store Write128/1
  Data Store Read129/1 -> Bitwise Operator130/1
  Bitwise Operator130/1 -> Data Store Write129/1
  Data Store Read130/1 -> Bitwise Operator131/1
  Bitwise Operator131/1 -> Data Store Write130/1
  Data Store Read131/1 -> Bitwise Operator132/1
  Bitwise Operator132/1 -> Data Store Write131/1
  Data Store Read132/1 -> Bitwise Operator133/1
  Bitwise Operator133/1 -> Data Store Write132/1
  Data Store Read133/1 -> Bitwise Operator134/1
  Bitwise Operator134/1 -> Data Store Write133/1
  Data Store Read134/1 -> Bitwise Operator135/1
  Bitwise Operator135/1 -> Data Store Write134/1
  Data Store Read135/1 -> Bitwise Operator136/1
  Bitwise Operator136/1 -> Data Store Write135/1
  Data Store Read136/1 -> Bitwise Operator137/1
  Bitwise Operator137/1 -> Data Store Write136/1
  Data Store Read137/1 -> Bitwise Operator138/1
  Bitwise Operator138/1 -> Data Store Write137/1
  Data Store Read138/1 -> Bitwise Operator139/1
  Bitwise Operator139/1 -> Data Store Write138/1
  Data Store Read139/1 -> Bitwise Operator140/1
  Bitwise Operator140/1 -> Data Store Write139/1
  Data Store Read140/1 -> Bitwise Operator141/1
  Bitwise Operator141/1 -> Data Store Write140/1
  Data Store Read141/1 -> Bitwise Operator142/1
  Bitwise Operator142/1 -> Data Store Write141/1
  Data Store Read142/1 -> Bitwise Operator143/1
  Bitwise Operator143/1 -> Data Store Write142/1
  Data Store Read143/1 -> Bitwise Operator144/1
  Bitwise Operator144/1 -> Data Store Write143/1
  Data Store Read144/1 -> Bitwise Operator145/1
  Bitwise Operator145/1 -> Data Store Write144/1
  Data Store Read145/1 -> Bitwise Operator146/1
  Bitwise Operator146/1 -> Data Store Write145/1
  Data Store Read146/1 -> Bitwise Operator147/1
  Bitwise Operator147/1 -> Data Store Write146/1
  Data Store Read147/1 -> Bitwise Operator148/1
  Bitwise Operator148/1 -> Data Store Write147/1
  Data Store Read148/1 -> Bitwise Operator149/1
  Bitwise Operator149/1 -> Data Store Write148/1
  Data Store Read149/1 -> Bitwise Operator150/1
  Bitwise Operator150/1 -> Data Store Write149/1
  Data Store Read150/1 -> Bitwise Operator151/1
  Bitwise Operator151/1 -> Data Store Write150/1
  Data Store Read151/1 -> Bitwise Operator152/1
  Bitwise Operator152/1 -> Data Store Write151/1
  Data Store Read152/1 -> Bitwise Operator153/1
  Bitwise Operator153/1 -> Data Store Write152/1
  Data Store Read153/1 -> Bitwise Operator154/1
  Bitwise Operator154/1 -> Data Store Write153/1
  Data Store Read154/1 -> Bitwise Operator155/1
  Bitwise Operator155/1 -> Data Store Write154/1
  Data Store Read155/1 -> Bitwise Operator156/1
  Bitwise Operator156/1 -> Data Store Write155/1
